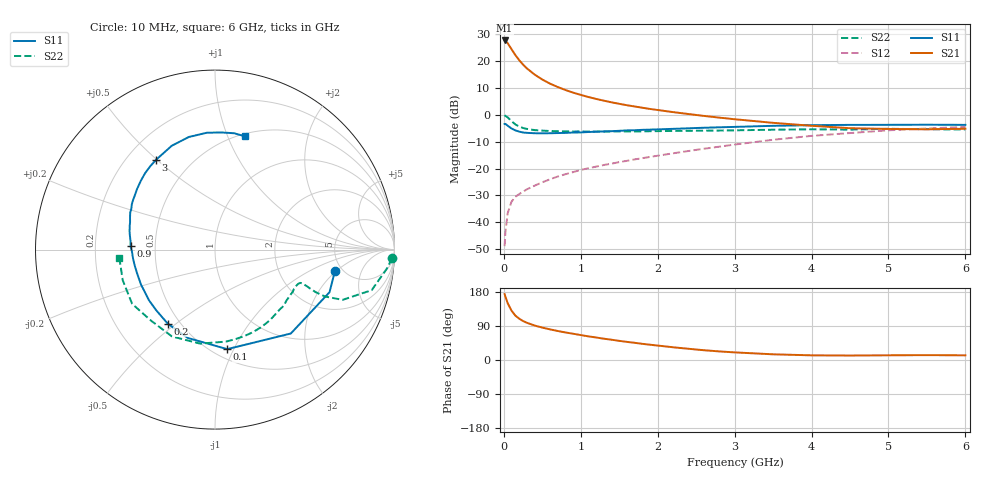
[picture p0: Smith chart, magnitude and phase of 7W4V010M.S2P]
! Infineon Technologies  Discrete & RF Semiconductors
! BFS17W
! Si NPN RF Bipolar Junction Transistor in SOT323
! VCE = 4 V  IC = 10 mA
! Common Emitter S-Parameters:  August  1999
# GHz  S  MA  R  50
!  f  S11  S21  S12  S22
! GHz  MAG  ANG  MAG  ANG  MAG  ANG  MAG  ANG
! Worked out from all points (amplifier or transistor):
!   36 points, 10 MHz to 6 GHz, reference 50 ohm
!   highest |S21| = 27.7 dB at 10 MHz (marker M1)
!   |S21| within 3 dB of that: start of sweep to 94.31 MHz
!   unconditionally stable (mu >= 1): 397.8 MHz to 2.415 GHz; 4.897 GHz to end of sweep
!   at 250 MHz: K = 0.79, MSG = 23.7 dB, |S12| = -28.6 dB
!   at 1.4 GHz: K = 1.20, MAG = 8.7 dB, |S12| = -18.1 dB
!   at 6 GHz: K = 1.06, MAG = -1.9 dB, |S12| = -4.5 dB
!   S11 on the Smith chart (normalised r, x): 10 MHz: 4.33, -1.93; 100 MHz: 0.58, -0.94; 200 MHz: 0.43, -0.47; 900 MHz: 0.36, +0.02; 3 GHz: 0.32, +0.50; 6 GHz: 0.52, +1.15
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0.01  0.6787 -10.2  24.35 173.9  0.0036 83.4  0.9884 -2.8
0.02  0.6808 -20.4  23.96 167.2  0.0065 88.1  0.9618 -6.5
0.05  0.6301 -47.9  21.62 150.1  0.0148 71.2  0.9019 -14.5
0.1  0.5587 -83.0  16.74 130.1  0.0243 58.7  0.764 -21.5
0.15  0.5151 -107.2  13 117.1  0.0299 53.7  0.6653 -23.1
0.2  0.4893 -122.6  10.45 109.0  0.0336 54.0  0.6077 -22.9
0.25  0.4706 -134.2  8.645 102.8  0.0373 54.2  0.5704 -22.2
0.3  0.4637 -142.6  7.346 98.2  0.0412 56.0  0.5494 -21.7
0.4  0.4559 -154.8  5.639 90.9  0.0482 57.5  0.5217 -21.2
0.5  0.4538 -163.0  4.563 85.5  0.0557 60.5  0.51 -21.3
0.6  0.4562 -169.0  3.822 80.8  0.0633 62.1  0.5022 -22.2
0.7  0.4595 -174.0  3.31 76.6  0.0713 63.6  0.4973 -23.4
0.9  0.4707 177.8  2.602 69.3  0.0861 65.5  0.4914 -26.8
1.1  0.481 170.5  2.154 62.3  0.1017 66.2  0.4902 -30.8
1.3  0.4933 164.4  1.842 56.2  0.1169 67.1  0.4889 -35.5
1.6  0.5155 156.4  1.515 47.8  0.1397 68.1  0.491 -42.8
2.2  0.5504 142.0  1.128 33.6  0.1928 69.1  0.503 -59.5
3  0.5985 123.3  0.831 20.1  0.2803 66.4  0.5163 -83.2
3.5  0.6268 112.6  0.712 15.0  0.3445 62.4  0.5304 -99.1
4.5  0.6527 94.0  0.566 11.8  0.4596 50.1  0.5327 -132.2
5.5  0.657 80.6  0.54 12.9  0.5588 37.3  0.5416 -161.7
6  0.6528 75.3  0.553 12.3  0.5981 31.1  0.5349 -174.7
